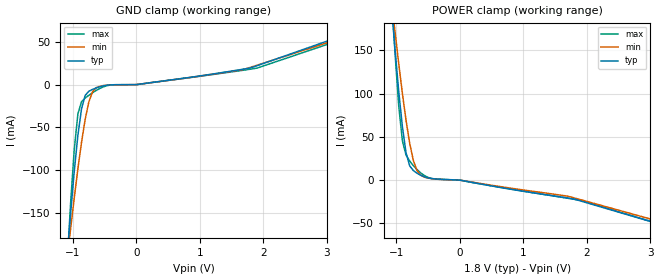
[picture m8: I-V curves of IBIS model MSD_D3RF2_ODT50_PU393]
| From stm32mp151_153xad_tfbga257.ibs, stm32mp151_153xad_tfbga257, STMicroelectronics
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[Model] MSD_D3RF2_ODT50_PU393
Model_type   Input
C_comp 2.254pF   2.216pF   2.282pF
Vinh = 1.150V
Vinl = 650.000mV
[Model Spec]
Vinh   1.150V   1.100V   1.200V
Vinl   650.000mV   600.000mV   700.000mV
[Temperature Range]   25.000   125.000   -40.000
[Voltage Range]   1.800V   1.700V   1.900V
[GND Clamp Reference]   0.00V   0.00V   0.00V
[POWER Clamp Reference]   1.800V   1.700V   1.900V
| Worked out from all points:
|   GND clamp passes 1 mA (typ) near -0.48 V on its own axis
|   POWER clamp passes 1 mA (typ) near -0.31 V on its own axis
[GND Clamp]
-1.785V   -919mA     -679.5mA   -1.289A
-1.094V   -204.7mA   -206.1mA   -214.8mA
-1.036V   -151mA     -168.8mA   -139.4mA
-978.8mV  -101.8mA   -132.9mA   -76.5mA
-921.2mV  -59.6mA    -98.67mA   -34.41mA
-863.6mV  -28.3mA    -67.44mA   -19.94mA
-806.1mV  -12.62mA   -40.6mA    -15.64mA
-748.5mV  -7.758mA   -20.27mA   -12.45mA
-690.9mV  -5.572mA   -8.4mA     -9.508mA
-575.8mV  -2.52mA    -1.89mA    -4.46mA
1.785V    19.34mA    19.93mA    17.93mA
3.57V     65.55mA    62.33mA    61.11mA
[Power Clamp]
-1.77V    920.7mA    688.7mA    1.287A
-1.079V   202.5mA    208.9mA    217.4mA
-1.021V   150.2mA    171.2mA    146.1mA
-963.6mV  102.8mA    134.8mA    85.89mA
-906.1mV  61.92mA    100.4mA    45.62mA
-848.5mV  31.57mA    69.14mA    28.93mA
-790.9mV  16.49mA    42.59mA    22.03mA
-733.3mV  11.03mA    22.73mA    16.76mA
-618.2mV  5.612mA    5.648mA    8.342mA
-445.5mV  1.796mA    1.654mA    1.795mA
1.8V      -22mA      -20.64mA   -22.26mA
3.585V    -60.56mA   -56.91mA   -60.53mA
